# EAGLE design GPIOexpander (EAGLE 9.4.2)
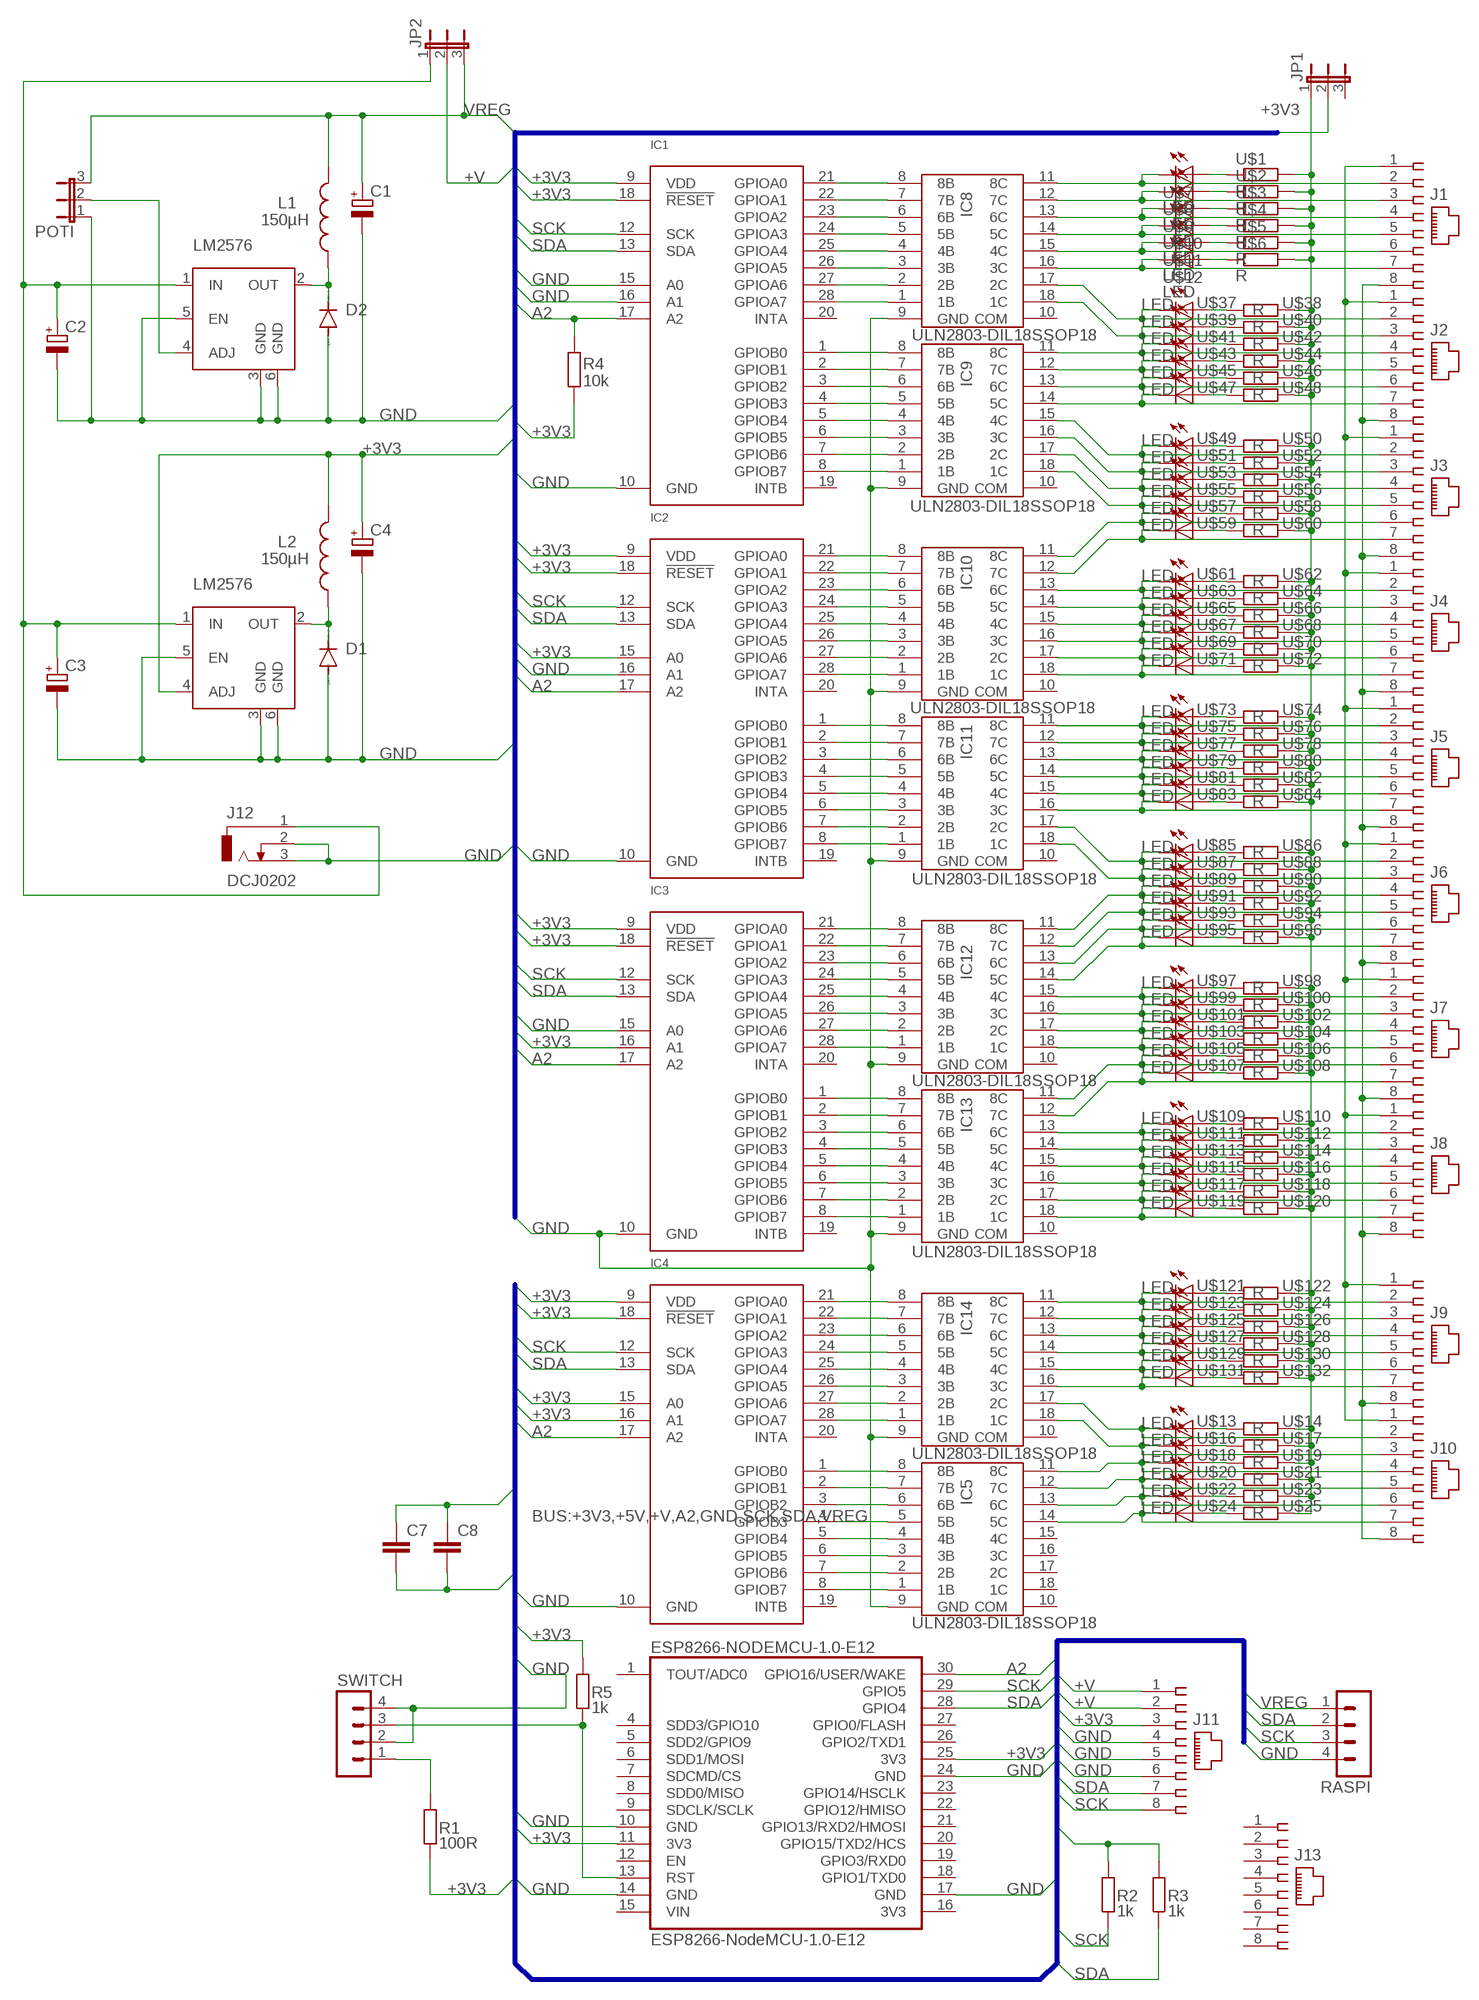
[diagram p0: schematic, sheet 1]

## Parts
C1  CPOL-EUE5-10.5  [E5-10,5]
C2  CPOL-EUE5-10.5  [E5-10,5]
C3  CPOL-EUE5-10.5  [E5-10,5]
C4  CPOL-EUE5-10.5  [E5-10,5]
C7  C-EUC0805  [C0805]
C8  C-EUC0805  [C0805]
D1  DIODE-SMB  [SMB]
D2  DIODE-SMB  [SMB]
ESP8266-NODEMCU-1.0-E12  ESP8266-NodeMCU-1.0-E12  MCP8266-MODULE  [MCP8266-MODULE]
IC1  MCP23017-DIL28-3SSOP28  [SO28W]
IC2  MCP23017-DIL28-3SSOP28  [SO28W]
IC3  MCP23017-DIL28-3SSOP28  [SO28W]
IC4  MCP23017-DIL28-3SSOP28  [SO28W]
IC5  ULN2803-DIL18SSOP18  [SO18W]
IC8  ULN2803-DIL18SSOP18  [SO18W]
IC9  ULN2803-DIL18SSOP18  [SO18W]
IC10  ULN2803-DIL18SSOP18  [SO18W]
IC11  ULN2803-DIL18SSOP18  [SO18W]
IC12  ULN2803-DIL18SSOP18  [SO18W]
IC13  ULN2803-DIL18SSOP18  [SO18W]
IC14  ULN2803-DIL18SSOP18  [SO18W]
J1  215877-7  [215877-7]
J2  215877-7  [215877-7]
J3  215877-7  [215877-7]
J4  215877-7  [215877-7]
J5  215877-7  [215877-7]
J6  215877-7  [215877-7]
J7  215877-7  [215877-7]
J8  215877-7  [215877-7]
J9  215877-7  [215877-7]
J10  215877-7  [215877-7]
J11  215877-7  [215877-7]
J12  DCJ0202  [DCJ0303]
J13  215877-7  [215877-7]
JP1  JP2E  [JP2]
JP2  JP2E  [JP2]
L1  150µH  BIG_COILS  [BIG_COIL]
L2  150µH  BIG_COILS  [BIG_COIL]
POTI  JP2E  [JP2]
R1  100R  R  [C0805]
R2  1k  R  [C0805]
R3  1k  R  [C0805]
R4  10k  R  [C0805]
R5  1k  R  [C0805]
RASPI  MA04-1  [MA04-1]
SWITCH  MA04-1  [MA04-1]
U$1  R  [C0805]
U$2  R  [C0805]
U$3  R  [C0805]
U$4  R  [C0805]
U$5  R  [C0805]
U$6  R  [C0805]
U$7  LED  [C0805]
U$8  LED  [C0805]
U$9  LED  [C0805]
U$10  LED  [C0805]
U$11  LED  [C0805]
U$12  LED  [C0805]
U$13  LED  [C0805]
U$14  R  [C0805]
U$16  LED  [C0805]
U$17  R  [C0805]
U$18  LED  [C0805]
U$19  R  [C0805]
U$20  LED  [C0805]
U$21  R  [C0805]
U$22  LED  [C0805]
U$23  R  [C0805]
U$24  LED  [C0805]
U$25  R  [C0805]
U$26  LM2576  [D2PAK]
U$28  LM2576  [D2PAK]
U$37  LED  [C0805]
U$38  R  [C0805]
U$39  LED  [C0805]
U$40  R  [C0805]
U$41  LED  [C0805]
U$42  R  [C0805]
U$43  LED  [C0805]
U$44  R  [C0805]
U$45  LED  [C0805]
U$46  R  [C0805]
U$47  LED  [C0805]
U$48  R  [C0805]
U$49  LED  [C0805]
U$50  R  [C0805]
U$51  LED  [C0805]
U$52  R  [C0805]
U$53  LED  [C0805]
U$54  R  [C0805]
U$55  LED  [C0805]
U$56  R  [C0805]
U$57  LED  [C0805]
U$58  R  [C0805]
U$59  LED  [C0805]
U$60  R  [C0805]
U$61  LED  [C0805]
U$62  R  [C0805]
U$63  LED  [C0805]
U$64  R  [C0805]
U$65  LED  [C0805]
U$66  R  [C0805]
U$67  LED  [C0805]
U$68  R  [C0805]
U$69  LED  [C0805]
U$70  R  [C0805]
U$71  LED  [C0805]
U$72  R  [C0805]
U$73  LED  [C0805]
U$74  R  [C0805]
U$75  LED  [C0805]
U$76  R  [C0805]
U$77  LED  [C0805]
U$78  R  [C0805]
U$79  LED  [C0805]
U$80  R  [C0805]
U$81  LED  [C0805]
U$82  R  [C0805]
U$83  LED  [C0805]
U$84  R  [C0805]
U$85  LED  [C0805]
U$86  R  [C0805]
U$87  LED  [C0805]
U$88  R  [C0805]
U$89  LED  [C0805]
U$90  R  [C0805]
U$91  LED  [C0805]
U$92  R  [C0805]
U$93  LED  [C0805]
U$94  R  [C0805]
U$95  LED  [C0805]
U$96  R  [C0805]
U$97  LED  [C0805]
U$98  R  [C0805]
U$99  LED  [C0805]
U$100  R  [C0805]
U$101  LED  [C0805]
U$102  R  [C0805]
U$103  LED  [C0805]
U$104  R  [C0805]
U$105  LED  [C0805]
U$106  R  [C0805]
U$107  LED  [C0805]
U$108  R  [C0805]
U$109  LED  [C0805]
U$110  R  [C0805]
U$111  LED  [C0805]
U$112  R  [C0805]
U$113  LED  [C0805]
U$114  R  [C0805]
U$115  LED  [C0805]
U$116  R  [C0805]
U$117  LED  [C0805]
U$118  R  [C0805]
U$119  LED  [C0805]
U$120  R  [C0805]
U$121  LED  [C0805]
U$122  R  [C0805]
U$123  LED  [C0805]
U$124  R  [C0805]
U$125  LED  [C0805]
U$126  R  [C0805]
U$127  LED  [C0805]
U$128  R  [C0805]
U$129  LED  [C0805]
U$130  R  [C0805]
U$131  LED  [C0805]
U$132  R  [C0805]

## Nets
+3V3: C4.+ C7.1 C8.1 ESP8266-NODEMCU-1.0-E12.11(3V3) ESP8266-NODEMCU-1.0-E12.25(3V3) IC1.9(VDD) IC1.18(!RESET) IC2.9(VDD) IC2.15(A0) IC2.18(!RESET) IC3.9(VDD) IC3.16(A1) IC3.18(!RESET) IC4.9(VDD) IC4.15(A0) IC4.16(A1) IC4.18(!RESET) J11.3 JP1.2 L2.P$2 R1.1 R2.2 R3.2 R4.1 R5.2 U$28.4(ADJ)
+V: J1.1 J2.1 J3.1 J4.1 J5.1 J6.1 J7.1 J8.1 J9.1 J10.1 J11.1 J11.2 JP2.2
A2: ESP8266-NODEMCU-1.0-E12.30(GPIO16/USER/WAKE) IC1.17(A2) IC2.17(A2) IC3.17(A2) IC4.17(A2) R4.2
GND: C1.- C2.- C3.- C4.- C7.2 C8.2 D1.A D2.A ESP8266-NODEMCU-1.0-E12.10(GND) ESP8266-NODEMCU-1.0-E12.14(GND) ESP8266-NODEMCU-1.0-E12.17(GND) ESP8266-NODEMCU-1.0-E12.24(GND) IC1.10(GND) IC1.15(A0) IC1.16(A1) IC2.10(GND) IC2.16(A1) IC3.10(GND) IC3.15(A0) IC4.10(GND) IC5.9(GND) IC8.9(GND) IC9.9(GND) IC10.9(GND) IC11.9(GND) IC12.9(GND) IC13.9(GND) IC14.9(GND) J1.8 J2.8 J3.8 J4.8 J5.8 J6.8 J7.8 J8.8 J9.8 J10.8 J11.4 J11.5 J11.6 J12.2 J12.3 POTI.1 RASPI.4 SWITCH.2 SWITCH.4 U$26.3(GND) U$26.5(EN) U$26.6(GND) U$28.3(GND) U$28.5(EN) U$28.6(GND)
N$1: IC1.21(GPIOA0) IC8.8(8B)
N$2: IC1.22(GPIOA1) IC8.7(7B)
N$3: IC1.23(GPIOA2) IC8.6(6B)
N$4: IC1.24(GPIOA3) IC8.5(5B)
N$5: IC1.25(GPIOA4) IC8.4(4B)
N$6: IC1.26(GPIOA5) IC8.3(3B)
N$7: IC1.27(GPIOA6) IC8.2(2B)
N$8: IC1.28(GPIOA7) IC8.1(1B)
N$9: IC4.8(GPIOB7) IC5.1(1B)
N$10: IC1.1(GPIOB0) IC9.8(8B)
N$11: IC1.2(GPIOB1) IC9.7(7B)
N$12: IC1.3(GPIOB2) IC9.6(6B)
N$13: IC1.4(GPIOB3) IC9.5(5B)
N$14: IC1.5(GPIOB4) IC9.4(4B)
N$15: IC1.6(GPIOB5) IC9.3(3B)
N$16: IC1.7(GPIOB6) IC9.2(2B)
N$17: IC1.8(GPIOB7) IC9.1(1B)
N$18: IC4.7(GPIOB6) IC5.2(2B)
N$19: IC2.21(GPIOA0) IC10.8(8B)
N$20: IC2.22(GPIOA1) IC10.7(7B)
N$21: IC2.23(GPIOA2) IC10.6(6B)
N$22: IC2.24(GPIOA3) IC10.5(5B)
N$23: IC2.25(GPIOA4) IC10.4(4B)
N$24: IC2.26(GPIOA5) IC10.3(3B)
N$25: IC2.27(GPIOA6) IC10.2(2B)
N$26: IC2.28(GPIOA7) IC10.1(1B)
N$27: IC4.6(GPIOB5) IC5.3(3B)
N$28: IC2.1(GPIOB0) IC11.8(8B)
N$29: IC2.2(GPIOB1) IC11.7(7B)
N$30: IC2.3(GPIOB2) IC11.6(6B)
N$31: IC2.4(GPIOB3) IC11.5(5B)
N$32: IC2.5(GPIOB4) IC11.4(4B)
N$33: IC2.6(GPIOB5) IC11.3(3B)
N$34: IC2.7(GPIOB6) IC11.2(2B)
N$35: IC2.8(GPIOB7) IC11.1(1B)
N$36: IC9.15(4C) J3.2 U$49.2(C)
N$37: IC3.21(GPIOA0) IC12.8(8B)
N$38: IC3.22(GPIOA1) IC12.7(7B)
N$39: IC3.23(GPIOA2) IC12.6(6B)
N$40: IC3.24(GPIOA3) IC12.5(5B)
N$41: IC3.25(GPIOA4) IC12.4(4B)
N$42: IC3.26(GPIOA5) IC12.3(3B)
N$43: IC3.27(GPIOA6) IC12.2(2B)
N$44: IC3.28(GPIOA7) IC12.1(1B)
N$45: IC9.16(3C) J3.3 U$51.2(C)
N$46: IC3.1(GPIOB0) IC13.8(8B)
N$47: IC3.2(GPIOB1) IC13.7(7B)
N$48: IC3.3(GPIOB2) IC13.6(6B)
N$49: IC3.4(GPIOB3) IC13.5(5B)
N$50: IC3.5(GPIOB4) IC13.4(4B)
N$51: IC3.6(GPIOB5) IC13.3(3B)
N$52: IC3.7(GPIOB6) IC13.2(2B)
N$53: IC3.8(GPIOB7) IC13.1(1B)
N$54: IC9.17(2C) J3.4 U$53.2(C)
N$55: IC4.21(GPIOA0) IC14.8(8B)
N$56: IC4.22(GPIOA1) IC14.7(7B)
N$57: IC4.23(GPIOA2) IC14.6(6B)
N$58: IC4.24(GPIOA3) IC14.5(5B)
N$59: IC4.25(GPIOA4) IC14.4(4B)
N$60: IC4.26(GPIOA5) IC14.3(3B)
N$61: IC4.27(GPIOA6) IC14.2(2B)
N$62: IC4.28(GPIOA7) IC14.1(1B)
N$63: IC8.17(2C) J2.2 U$37.2(C)
N$64: IC4.5(GPIOB4) IC5.4(4B)
N$65: IC4.4(GPIOB3) IC5.5(5B)
N$66: IC4.3(GPIOB2) IC5.6(6B)
N$67: IC4.2(GPIOB1) IC5.7(7B)
N$68: IC4.1(GPIOB0) IC5.8(8B)
N$69: IC14.17(2C) J10.2 U$13.2(C)
N$70: JP1.1 U$1.2 U$2.2 U$3.2 U$4.2 U$5.2 U$6.2 U$14.2 U$17.2 U$19.2 U$21.2 U$23.2 U$25.2 U$38.2 U$40.2 U$42.2 U$44.2 U$46.2 U$48.2 U$50.2 U$52.2 U$54.2 U$56.2 U$58.2 U$60.2 U$62.2 U$64.2 U$66.2 U$68.2 U$70.2 U$72.2 U$74.2 U$76.2 U$78.2 U$80.2 U$82.2 U$84.2 U$86.2 U$88.2 U$90.2 U$92.2 U$94.2 U$96.2 U$98.2 U$100.2 U$102.2 U$104.2 U$106.2 U$108.2 U$110.2 U$112.2 U$114.2 U$116.2 U$118.2 U$120.2 U$122.2 U$124.2 U$126.2 U$128.2 U$130.2 U$132.2
N$71: D2.C L1.P$1 U$26.2(OUT)
N$72: IC8.11(8C) J1.2 U$7.2(C)
N$73: C2.+ C3.+ J12.1 JP2.1 U$26.1(IN) U$28.1(IN)
N$74: IC14.18(1C) J10.3 U$16.2(C)
N$75: IC5.11(8C) J10.4 U$18.2(C)
N$76: IC5.12(7C) J10.5 U$20.2(C)
N$77: IC5.13(6C) J10.6 U$22.2(C)
N$78: IC5.14(5C) J10.7 U$24.2(C)
N$79: U$13.1(A) U$14.1
N$80: U$16.1(A) U$17.1
N$81: IC8.18(1C) J2.3 U$39.2(C)
N$82: U$18.1(A) U$19.1
N$83: U$20.1(A) U$21.1
N$84: U$22.1(A) U$23.1
N$85: U$24.1(A) U$25.1
N$86: POTI.2 U$26.4(ADJ)
N$87: D1.C L2.P$1 U$28.2(OUT)
N$88: ESP8266-NODEMCU-1.0-E12.13(RST) R5.1 SWITCH.3
N$89: R1.2 SWITCH.1
N$90: IC9.12(7C) J2.5 U$43.2(C)
N$99: IC9.11(8C) J2.4 U$41.2(C)
N$128: IC9.18(1C) J3.5 U$55.2(C)
N$215: IC10.11(8C) J3.6 U$57.2(C)
N$217: IC8.12(7C) J1.3 U$8.2(C)
N$218: IC8.13(6C) J1.4 U$9.2(C)
N$223: IC9.13(6C) J2.6 U$45.2(C)
N$224: IC9.14(5C) J2.7 U$47.2(C)
N$225: IC8.14(5C) J1.5 U$10.2(C)
N$226: IC8.15(4C) J1.6 U$11.2(C)
N$228: IC8.16(3C) J1.7 U$12.2(C)
N$229: IC10.12(7C) J3.7 U$59.2(C)
N$230: IC10.13(6C) J4.2 U$61.2(C)
N$232: IC10.14(5C) J4.3 U$63.2(C)
N$233: IC10.15(4C) J4.4 U$65.2(C)
N$234: IC10.16(3C) J4.5 U$67.2(C)
N$235: IC10.17(2C) J4.6 U$69.2(C)
N$238: IC10.18(1C) J4.7 U$71.2(C)
N$239: IC11.14(5C) J5.5 U$79.2(C)
N$240: IC11.15(4C) J5.6 U$81.2(C)
N$241: IC11.16(3C) J5.7 U$83.2(C)
N$242: IC11.11(8C) J5.2 U$73.2(C)
N$243: IC11.12(7C) J5.3 U$75.2(C)
N$244: IC11.13(6C) J5.4 U$77.2(C)
N$245: IC11.17(2C) J6.2 U$85.2(C)
N$246: IC11.18(1C) J6.3 U$87.2(C)
N$247: IC12.11(8C) J6.4 U$89.2(C)
N$248: IC12.12(7C) J6.5 U$91.2(C)
N$249: IC12.13(6C) J6.6 U$93.2(C)
N$250: IC12.14(5C) J6.7 U$95.2(C)
N$251: IC12.15(4C) J7.2 U$97.2(C)
N$252: IC12.16(3C) J7.3 U$99.2(C)
N$253: IC12.17(2C) J7.4 U$101.2(C)
N$254: IC12.18(1C) J7.5 U$103.2(C)
N$255: IC13.11(8C) J7.6 U$105.2(C)
N$256: IC13.12(7C) J7.7 U$107.2(C)
N$257: IC13.13(6C) J8.2 U$109.2(C)
N$258: IC13.14(5C) J8.3 U$111.2(C)
N$259: IC13.15(4C) J8.4 U$113.2(C)
N$260: IC13.16(3C) J8.5 U$115.2(C)
N$261: IC13.17(2C) J8.6 U$117.2(C)
N$262: IC13.18(1C) J8.7 U$119.2(C)
N$263: IC14.11(8C) J9.2 U$121.2(C)
N$264: IC14.12(7C) J9.3 U$123.2(C)
N$265: IC14.13(6C) J9.4 U$125.2(C)
N$266: IC14.14(5C) J9.5 U$127.2(C)
N$267: IC14.15(4C) J9.6 U$129.2(C)
N$268: IC14.16(3C) J9.7 U$131.2(C)
N$329: U$1.1 U$7.1(A)
N$330: U$2.1 U$8.1(A)
N$331: U$3.1 U$9.1(A)
N$332: U$4.1 U$10.1(A)
N$333: U$5.1 U$11.1(A)
N$334: U$6.1 U$12.1(A)
N$347: U$37.1(A) U$38.1
N$348: U$39.1(A) U$40.1
N$349: U$41.1(A) U$42.1
N$350: U$43.1(A) U$44.1
N$351: U$45.1(A) U$46.1
N$352: U$47.1(A) U$48.1
N$353: U$49.1(A) U$50.1
N$354: U$51.1(A) U$52.1
N$355: U$53.1(A) U$54.1
N$356: U$55.1(A) U$56.1
N$357: U$57.1(A) U$58.1
N$358: U$59.1(A) U$60.1
N$359: U$61.1(A) U$62.1
N$360: U$63.1(A) U$64.1
N$361: U$65.1(A) U$66.1
N$362: U$67.1(A) U$68.1
N$363: U$69.1(A) U$70.1
N$364: U$71.1(A) U$72.1
N$365: U$73.1(A) U$74.1
N$366: U$75.1(A) U$76.1
N$367: U$77.1(A) U$78.1
N$368: U$79.1(A) U$80.1
N$369: U$81.1(A) U$82.1
N$370: U$83.1(A) U$84.1
N$371: U$85.1(A) U$86.1
N$372: U$87.1(A) U$88.1
N$373: U$89.1(A) U$90.1
N$374: U$91.1(A) U$92.1
N$375: U$93.1(A) U$94.1
N$376: U$95.1(A) U$96.1
N$377: U$97.1(A) U$98.1
N$378: U$99.1(A) U$100.1
N$379: U$101.1(A) U$102.1
N$380: U$103.1(A) U$104.1
N$381: U$105.1(A) U$106.1
N$382: U$107.1(A) U$108.1
N$383: U$109.1(A) U$110.1
N$384: U$111.1(A) U$112.1
N$385: U$113.1(A) U$114.1
N$386: U$115.1(A) U$116.1
N$387: U$117.1(A) U$118.1
N$388: U$119.1(A) U$120.1
N$389: U$121.1(A) U$122.1
N$390: U$123.1(A) U$124.1
N$391: U$125.1(A) U$126.1
N$392: U$127.1(A) U$128.1
N$393: U$129.1(A) U$130.1
N$394: U$131.1(A) U$132.1
SCK: ESP8266-NODEMCU-1.0-E12.29(GPIO5) IC1.12(SCK) IC2.12(SCK) IC3.12(SCK) IC4.12(SCK) J11.8 R2.1 RASPI.3
SDA: ESP8266-NODEMCU-1.0-E12.28(GPIO4) IC1.13(SDA) IC2.13(SDA) IC3.13(SDA) IC4.13(SDA) J11.7 R3.1 RASPI.2
VREG: C1.+ JP2.3 L1.P$2 POTI.3 RASPI.1
Unconnected: ESP8266-NODEMCU-1.0-E12.1(TOUT/ADC0) ESP8266-NODEMCU-1.0-E12.4(SDD3/GPIO10) ESP8266-NODEMCU-1.0-E12.5(SDD2/GPIO9) ESP8266-NODEMCU-1.0-E12.6(SDD1/MOSI) ESP8266-NODEMCU-1.0-E12.7(SDCMD/CS) ESP8266-NODEMCU-1.0-E12.8(SDD0/MISO) ESP8266-NODEMCU-1.0-E12.9(SDCLK/SCLK) ESP8266-NODEMCU-1.0-E12.12(EN) ESP8266-NODEMCU-1.0-E12.15(VIN) ESP8266-NODEMCU-1.0-E12.16(3V3) ESP8266-NODEMCU-1.0-E12.18(GPIO1/TXD0) ESP8266-NODEMCU-1.0-E12.19(GPIO3/RXD0) ESP8266-NODEMCU-1.0-E12.20(GPIO15/TXD2/HCS) ESP8266-NODEMCU-1.0-E12.21(GPIO13/RXD2/HMOSI) ESP8266-NODEMCU-1.0-E12.22(GPIO12/HMISO) ESP8266-NODEMCU-1.0-E12.23(GPIO14/HSCLK) ESP8266-NODEMCU-1.0-E12.26(GPIO2/TXD1) ESP8266-NODEMCU-1.0-E12.27(GPIO0/FLASH) IC1.19(INTB) IC1.20(INTA) IC2.19(INTB) IC2.20(INTA) IC3.19(INTB) IC3.20(INTA) IC4.19(INTB) IC4.20(INTA) IC5.10(COM) IC5.15(4C) IC5.16(3C) IC5.17(2C) IC5.18(1C) IC8.10(COM) IC9.10(COM) IC10.10(COM) IC11.10(COM) IC12.10(COM) IC13.10(COM) IC14.10(COM) J13.1 J13.2 J13.3 J13.4 J13.5 J13.6 J13.7 J13.8 JP1.3

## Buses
BUS:+3V3,+5V,+V,A2,GND,SCK,SDA,VREG

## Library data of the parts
C1-C4 = rcl:CPOL-EU: POLARIZED CAPACITOR, European symbol; SPICEPREFIX: C
C7 C8 = rcl:C-EU: CAPACITOR, European symbol; SPICEPREFIX: C
D1 D2 = diode:DIODE-: DIODE
ESP8266-NODEMCU-1.0-E12 = GPIOexpander:MCP8266-MODULE
IC1 = GPIOexpander:MCP23017-DIL28-3: GPIO expander; SPICEPREFIX: X
IC2-IC4 = GPIOexpander:MCP23017-DIL28-3: GPIO expander
IC5 IC8-IC14 = GPIOexpander:ULN2803-DIL18
J1-J11 J13 = con-amp:215877-7: AMP connector
J12 = GPIOexpander:DCJ0202: DC POWER JACK Source: DCJ0202.pdf
JP1 JP2 POTI = jumper-alex:JP2E: JUMPER
L1 L2 = GPIOexpander:BIG_COILS
R1-R5 U$1-U$6 U$14 U$17 U$19 U$21 U$23 U$25 U$38 U$40 U$42 U$44 U$46 U$48 U$50 U$52 U$54 U$56 U$58 U$60 U$62 U$64 U$66 U$68 U$70 U$72 U$74 U$76 U$78 U$80 U$82 U$84 U$86 U$88 U$90 U$92 U$94 U$96 U$98 U$100 U$102 U$104 U$106 U$108 U$110 U$112 U$114 U$116 U$118 U$120 U$122 U$124 U$126 U$128 U$130 U$132 = GPIOexpander:R
RASPI SWITCH = con-lstb:MA04-1: PIN HEADER; OC_FARNELL: unknown; OC_NEWARK: unknown
U$7-U$13 U$16 U$18 U$20 U$22 U$24 U$37 U$39 U$41 U$43 U$45 U$47 U$49 U$51 U$53 U$55 U$57 U$59 U$61 U$63 U$65 U$67 U$69 U$71 U$73 U$75 U$77 U$79 U$81 U$83 U$85 U$87 U$89 U$91 U$93 U$95 U$97 U$99 U$101 U$103 U$105 U$107 U$109 U$111 U$113 U$115 U$117 U$119 U$121 U$123 U$125 U$127 U$129 U$131 = GPIOexpander:LED
U$26 U$28 = GPIOexpander:LM2576

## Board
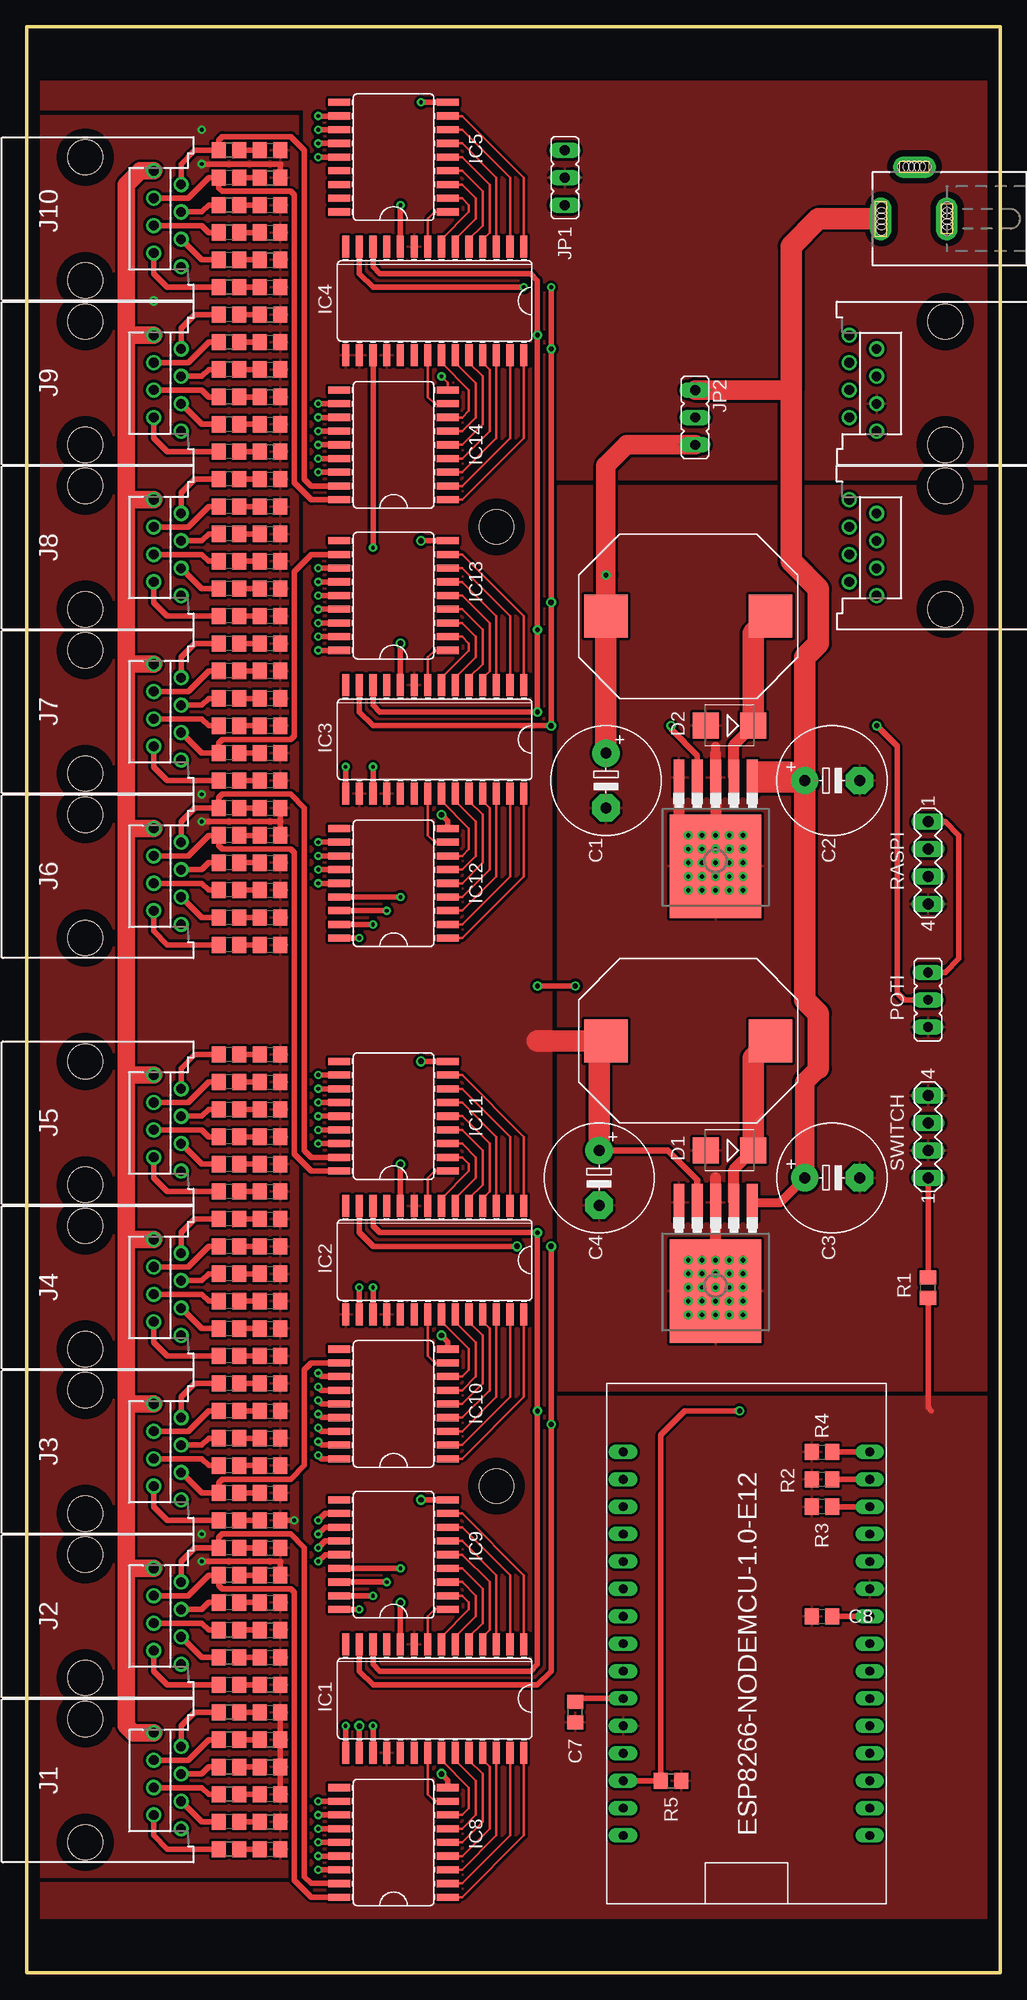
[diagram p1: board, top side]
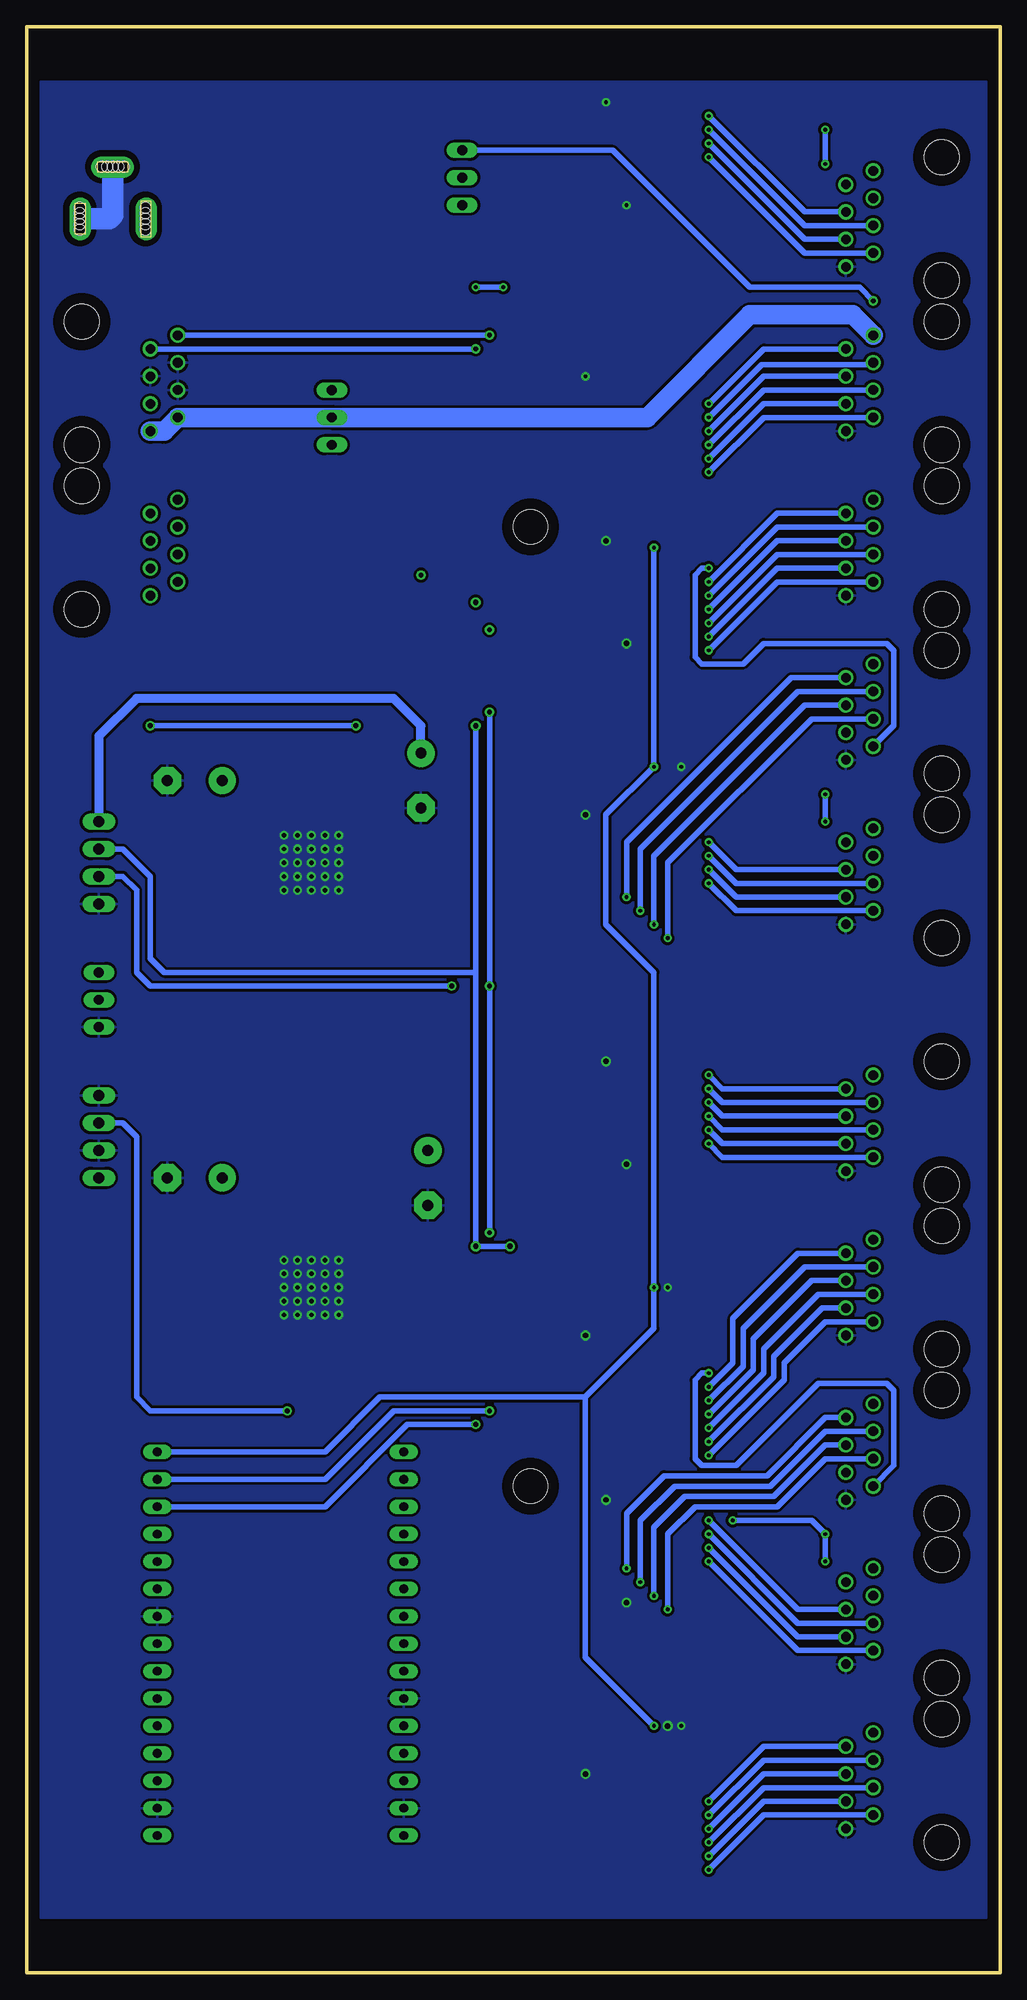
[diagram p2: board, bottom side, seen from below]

Size 90.17 x 180.34 mm. Coordinates in mm from the lower left corner, seen from the top.
Outline: 0,0 90.17,0 90.17,180.34 0,180.34 0,0
Copper layers (1*16): Top 0.035mm / dielectric 1.5mm / Bottom 0.035mm
Design rules "default": minimum track width 6mil, minimum drill 0.35mm, track to track 6mil, track to pad 6mil, pad to pad 6mil, via to via 6mil, smd to smd 6mil, copper to edge 40mil, drill to drill 6mil, minimum pad ring 10mil, minimum via ring 8mil, stop-mask expansion 4mil, vias tented up to drill 0mil, thermal gap 10mil
Holes 3.2 mm at 43.5,133.99 43.5,45.09

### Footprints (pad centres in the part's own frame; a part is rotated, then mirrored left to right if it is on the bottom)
E5-10,5 = drill 1.016 pad 2.54: + -2.54,0 | drill 1.016 pad 2.54 octagon: - 2.54,0
C0805 = smd 1.3 x 1.5: 1 -0.95,0; 2 0.95,0
SMB = smd 2.4 x 2.4: A 2.2,0; C -2.2,0
MCP8266-MODULE = drill 0.813 long: 1 41.91,24.13; 2 39.37,24.13; 3 36.83,24.13; 4 34.29,24.13; 5 31.75,24.13; 6 29.21,24.13; 7 26.67,24.13; 8 24.13,24.13; 9 21.59,24.13; 10 19.05,24.13; 11 16.51,24.13; 12 13.97,24.13; 13 11.43,24.13; 14 8.89,24.13; 15 6.35,24.13; 16 6.35,1.27; 17 8.89,1.27; 18 11.43,1.27; 19 13.97,1.27; 20 16.51,1.27; 21 19.05,1.27; 22 21.59,1.27; 23 24.13,1.27; 24 26.67,1.27; 25 29.21,1.27; 26 31.75,1.27; 27 34.29,1.27; 28 36.83,1.27; 29 39.37,1.27; 30 41.91,1.27
SO28W = smd 0.66 x 2.032: 1 -8.255,-5.029; 2 -6.985,-5.029; 3 -5.715,-5.029; 4 -4.445,-5.029; 5 -3.175,-5.029; 6 -1.905,-5.029; 7 -0.635,-5.029; 8 0.635,-5.029; 9 1.905,-5.029; 10 3.175,-5.029; 11 4.445,-5.029; 12 5.715,-5.029; 13 6.985,-5.029; 14 8.255,-5.029; 15 8.255,5.029; 16 6.985,5.029; 17 5.715,5.029; 18 4.445,5.029; 19 3.175,5.029; 20 1.905,5.029; 21 0.635,5.029; 22 -0.635,5.029; 23 -1.905,5.029; 24 -3.175,5.029; 25 -4.445,5.029; 26 -5.715,5.029; 27 -6.985,5.029; 28 -8.255,5.029
SO18W = smd 0.66 x 2.032: 1 -5.715,-5.029; 2 -4.445,-5.029; 3 -3.175,-5.029; 4 -1.905,-5.029; 5 -0.635,-5.029; 6 0.635,-5.029; 7 1.905,-5.029; 8 3.175,-5.029; 9 4.445,-5.029; 10 4.445,5.029; 11 3.175,5.029; 12 1.905,5.029; 13 0.635,5.029; 14 -0.635,5.029; 15 -1.905,5.029; 16 -3.175,5.029; 17 -4.445,5.029; 18 -5.715,5.029
215877-7 = drill 0.889: 1 -4.445,6.35; 2 -3.175,8.89; 3 -1.905,6.35; 4 -0.635,8.89; 5 0.635,6.35; 6 1.905,8.89; 7 3.175,6.35; 8 4.445,8.89 | hole 3.251: -5.715,0; 5.715,0
DCJ0303 = drill 1 pad 2 long: 1 0,3.1; 2 4.8,0; 3 0,-3 | hole 1: 0,3.048; 0.508,3.048; -0.508,3.048; -1.016,3.048; 1.016,3.048; 0,-3.048; 0.508,-3.048; 1.016,-3.048; -0.508,-3.048; -1.016,-3.048; 4.826,0; 4.826,0.508; 4.826,1.016; 4.826,-0.508; 4.826,-1.016
JP2 = drill 0.914 long: 1 -2.54,0; 2 0,0; 3 2.54,0
BIG_COIL = smd 4 x 4: P$1 15.24,0; P$2 0,0
MA04-1 = drill 1.016 long: 1 -3.81,0; 2 -1.27,0; 3 1.27,0; 4 3.81,0
D2PAK = smd 1 x 3.4: 1 -3.4,-7.875; 2 -1.7,-7.875; 3 0,-7.875; 4 1.7,-7.875; 5 3.4,-7.875 | smd 8.5 x 9.6: 6 0,0.325

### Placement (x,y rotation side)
C1  53.66,110.49 270 top
C2  74.61,110.49 0 top
C3  74.61,73.66 0 top
C4  53.02,73.66 270 top
C7  50.8,24.13 90 top
C8  73.66,33.02 0 top
D1  65.09,76.2 180 top
D2  65.09,115.57 180 top
ESP8266-NODEMCU-1.0-E12  79.38,6.35 90 top
IC1  37.78,25.4 180 top
IC2  37.78,66.04 180 top
IC3  37.78,114.3 180 top
IC4  37.78,154.94 180 top
IC5  33.97,168.91 90 top
IC8  33.97,12.7 90 top
IC9  33.97,39.37 90 top
IC10  33.97,53.34 90 top
IC11  33.97,80.01 90 top
IC12  33.97,101.6 90 top
IC13  33.97,128.27 90 top
IC14  33.97,142.24 90 top
J1  5.4,17.78 270 top
J2  5.4,33.02 270 top
J3  5.4,48.26 270 top
J4  5.4,63.5 270 top
J5  5.4,78.74 270 top
J6  5.4,101.6 270 top
J7  5.4,116.84 270 top
J8  5.4,132.08 270 top
J9  5.4,147.32 270 top
J10  5.4,162.56 270 top
J11  85.09,147.32 90 top
J12  82.23,162.56 90 top
J13  85.09,132.08 90 top
JP1  49.85,166.37 270 top
JP2  61.91,144.15 270 top
L1  53.66,125.73 0 top
L2  53.66,86.36 0 top
POTI  83.5,90.17 90 top
R1  83.5,63.5 90 top
R2  73.66,45.72 180 top
R3  73.66,43.18 180 top
R4  73.66,48.26 0 top
R5  59.69,17.78 0 top
RASPI  83.5,102.87 270 top
SWITCH  83.5,77.47 90 top
U$1  22.54,24.13 0 top
U$2  22.54,21.59 0 top
U$3  22.54,19.05 0 top
U$4  22.54,16.51 0 top
U$5  22.54,13.97 0 top
U$6  22.54,11.43 0 top
U$7  18.73,24.13 180 top
U$8  18.73,21.59 180 top
U$9  18.73,19.05 180 top
U$10  18.73,16.51 180 top
U$11  18.73,13.97 180 top
U$12  18.73,11.43 180 top
U$13  18.73,168.91 180 top
U$14  22.54,168.91 0 top
U$16  18.73,166.37 180 top
U$17  22.54,166.37 0 top
U$18  18.73,163.83 180 top
U$19  22.54,163.83 0 top
U$20  18.73,161.29 180 top
U$21  22.54,161.29 0 top
U$22  18.73,158.75 180 top
U$23  22.54,158.75 0 top
U$24  18.73,156.21 180 top
U$25  22.54,156.21 0 top
U$26  63.82,102.87 180 top
U$28  63.82,63.5 180 top
U$37  18.73,39.37 180 top
U$38  22.54,39.37 0 top
U$39  18.73,36.83 180 top
U$40  22.54,36.83 0 top
U$41  18.73,34.29 180 top
U$42  22.54,34.29 0 top
U$43  18.73,31.75 180 top
U$44  22.54,31.75 0 top
U$45  18.73,29.21 180 top
U$46  22.54,29.21 0 top
U$47  18.73,26.67 180 top
U$48  22.54,26.67 0 top
U$49  18.73,54.61 180 top
U$50  22.54,54.61 0 top
U$51  18.73,52.07 180 top
U$52  22.54,52.07 0 top
U$53  18.73,49.53 180 top
U$54  22.54,49.53 0 top
U$55  18.73,46.99 180 top
U$56  22.54,46.99 0 top
U$57  18.73,44.45 180 top
U$58  22.54,44.45 0 top
U$59  18.73,41.91 180 top
U$60  22.54,41.91 0 top
U$61  18.73,69.85 180 top
U$62  22.54,69.85 0 top
U$63  18.73,67.31 180 top
U$64  22.54,67.31 0 top
U$65  18.73,64.77 180 top
U$66  22.54,64.77 0 top
U$67  18.73,62.23 180 top
U$68  22.54,62.23 0 top
U$69  18.73,59.69 180 top
U$70  22.54,59.69 0 top
U$71  18.73,57.15 180 top
U$72  22.54,57.15 0 top
U$73  18.73,85.09 180 top
U$74  22.54,85.09 0 top
U$75  18.73,82.55 180 top
U$76  22.54,82.55 0 top
U$77  18.73,80.01 180 top
U$78  22.54,80.01 0 top
U$79  18.73,77.47 180 top
U$80  22.54,77.47 0 top
U$81  18.73,74.93 180 top
U$82  22.54,74.93 0 top
U$83  18.73,72.39 180 top
U$84  22.54,72.39 0 top
U$85  18.73,107.95 180 top
U$86  22.54,107.95 0 top
U$87  18.73,105.41 180 top
U$88  22.54,105.41 0 top
U$89  18.73,102.87 180 top
U$90  22.54,102.87 0 top
U$91  18.73,100.33 180 top
U$92  22.54,100.33 0 top
U$93  18.73,97.79 180 top
U$94  22.54,97.79 0 top
U$95  18.73,95.25 180 top
U$96  22.54,95.25 0 top
U$97  18.73,123.19 180 top
U$98  22.54,123.19 0 top
U$99  18.73,120.65 180 top
U$100  22.54,120.65 0 top
U$101  18.73,118.11 180 top
U$102  22.54,118.11 0 top
U$103  18.73,115.57 180 top
U$104  22.54,115.57 0 top
U$105  18.73,113.03 180 top
U$106  22.54,113.03 0 top
U$107  18.73,110.49 180 top
U$108  22.54,110.49 0 top
U$109  18.73,138.43 180 top
U$110  22.54,138.43 0 top
U$111  18.73,135.89 180 top
U$112  22.54,135.89 0 top
U$113  18.73,133.35 180 top
U$114  22.54,133.35 0 top
U$115  18.73,130.81 180 top
U$116  22.54,130.81 0 top
U$117  18.73,128.27 180 top
U$118  22.54,128.27 0 top
U$119  18.73,125.73 180 top
U$120  22.54,125.73 0 top
U$121  18.73,153.67 180 top
U$122  22.54,153.67 0 top
U$123  18.73,151.13 180 top
U$124  22.54,151.13 0 top
U$125  18.73,148.59 180 top
U$126  22.54,148.59 0 top
U$127  18.73,146.05 180 top
U$128  22.54,146.05 0 top
U$129  18.73,143.51 180 top
U$130  22.54,143.51 0 top
U$131  18.73,140.97 180 top
U$132  22.54,140.97 0 top

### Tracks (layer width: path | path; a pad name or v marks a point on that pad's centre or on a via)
+3V3
  Top 0.508: R1.1 83.5,52.39 83.82,52.07
  Top 0.61: U$28.4 62.12,73.45 59.37,76.2 C4.+
  Top 2: 47.31,86.36 L2.P$2 53.02,85.73 C4.+
  pour Top (isolate 0.254): 1.27,5.08 1.27,8.26 25.72,8.26 25.72,172.72 1.27,172.72 1.27,175.26 88.9,175.26 88.9,138.43 48.58,138.43 48.58,53.34 88.9,53.34 88.9,5.08
+V
  Top 1.27: 9.53,67.95 9.21,67.63
  Top 1.6: 9.21,37.47 9.21,52.71 | 9.21,52.71 9.21,67.63 9.21,83.19 | 9.21,83.19 9.21,106.05 | 9.21,106.05 9.21,121.28 | 9.21,121.28 9.21,136.53 | J2.1 9.21,37.47 | J3.1 9.21,52.71 | J4.1 9.53,67.95 | J5.1 9.21,83.19 | J6.1 9.21,106.05 | J7.1 9.21,121.28 | J8.1 9.21,136.53 | J1.1 9.84,22.22 9.21,22.86 9.21,37.47 | J10.1 10.48,167 9.21,165.74 9.21,151.77 | 9.21,136.53 9.21,151.77 | J9.1 9.21,151.77
  Bottom 1.8: J9.1 13.65,153.67 23.18,153.67 32.7,144.15 JP2.2 J11.2 77.47,142.88 J11.1
A2  (via drill 0.35)
  Top 0.508: v32.07,22.86 IC1.17 | IC3.17 v32.07,111.76 | IC2.17 v32.07,63.5 | v32.07,132.08 IC4.17 | R4.2 ESP8266-NODEMCU-1.0-E12.30
  Bottom 0.508: v32.07,22.86 38.42,29.21 38.42,53.34 | v32.07,132.08 v32.07,111.76 36.51,107.31 36.51,97.16 32.07,92.71 v32.07,63.5 32.07,59.69 38.42,53.34 | ESP8266-NODEMCU-1.0-E12.30 62.55,48.26 57.47,53.34 38.42,53.34
GND  (via drill 0.35, 0.4, 0.5)
  Top 0.254: IC14.9 39,147.37 v38.42,147.96
  Top 0.508: IC10.9 39,58.47 v38.42,59.05 | IC11.9 v36.51,84.45 | IC12.9 39,106.73 v38.42,107.31 | IC13.9 v36.51,132.72 | IC2.10 v34.61,74.93 | IC9.9 v36.51,43.82 | IC1.10 v34.61,34.29 | IC8.9 39,17.83 v38.42,18.41 | IC1.16 v30.8,22.86 | IC3.10 v34.61,123.19 | IC4.10 v34.61,163.83 | IC1.15 v29.53,22.86 | IC2.16 v30.8,63.5 | IC3.15 v29.53,111.76 | IC5.9 v36.51,173.35 | C7.2 51.12,25.4 ESP8266-NODEMCU-1.0-E12.10 | C8.2 ESP8266-NODEMCU-1.0-E12.24
  Top 0.813: 63.82,113.03 63.82,113.67
  Top 1.016: U$26.6 U$26.3 63.82,113.03 | U$26.5 60.42,105 v63.82,101.6 | U$28.6 63.82,73.66
  Bottom 2: J12.3 82.55,162.56 82.23,162.88 J12.2
  other vias: 63.82,102.87 62.55,102.87 65.09,102.87 65.09,101.6 62.55,101.6 62.55,104.14 63.82,104.14 65.09,104.14 65.09,100.33 63.82,100.33 62.55,100.33 61.28,100.33 61.28,101.6 61.28,102.87 61.28,104.14 61.28,105.41 62.55,105.41 63.82,105.41 65.09,105.41 66.36,105.41 66.36,104.14 66.36,102.87 66.36,101.6 66.36,100.33 63.82,63.5 61.28,66.04 66.36,66.04 66.36,60.96 61.28,60.96 63.82,60.96 63.82,66.04 66.36,63.5 61.28,63.5 61.28,64.77 61.28,62.23 62.55,60.96 65.09,60.96 66.36,62.23 66.36,64.77 65.09,66.04 62.55,66.04 62.55,64.77 62.55,63.5 62.55,62.23 63.82,62.23 65.09,62.23 65.09,63.5 65.09,64.77 63.82,64.77
  pour Bottom (isolate 0.254): 1.27,5.08 1.27,175.26 88.9,175.26 88.9,5.08
  pour Top (isolate 0.254): 88.9,137.8 49.21,137.8 49.21,53.98 88.9,53.98
N$1
  Top 0.254: IC1.21 37.15,16.51 37.78,15.88 IC8.8
N$2
  Top 0.203: IC1.22 38.42,19.68
  Top 0.254: 38.42,19.68 40.96,17.14 40.96,15.24 40.32,14.61 IC8.7
N$3
  Top 0.203: IC1.23 39.69,19.68
  Top 0.254: 39.69,19.68 41.59,17.78 41.59,14.61 40.32,13.34 IC8.6
N$4
  Top 0.203: IC1.24 40.96,19.68
  Top 0.254: 40.96,19.68 42.23,18.41 42.23,13.97 40.32,12.07 IC8.5
N$5
  Top 0.203: IC1.25 42.23,19.68
  Top 0.254: 42.23,19.68 42.86,19.05 42.86,13.34 40.32,10.79 IC8.4
N$6
  Top 0.254: IC1.26 43.5,12.7 40.32,9.53 IC8.3
N$7
  Top 0.254: IC1.27 44.77,12.7 40.32,8.26 IC8.2
N$8
  Top 0.254: IC1.28 46.04,12.7 40.32,6.98 IC8.1
N$9
  Top 0.254: IC5.1 37.78,163.19 37.15,162.56 IC4.8
N$10
  Top 0.254: IC1.1 46.04,36.83 40.32,42.55 IC9.8
N$11
  Top 0.254: IC1.2 44.77,36.83 40.32,41.28 IC9.7
N$12
  Top 0.254: IC1.3 43.5,36.83 40.32,40.01 IC9.6
N$13
  Top 0.203: IC1.4 42.23,31.11
  Top 0.254: 42.23,31.11 42.86,31.75 42.86,36.2 40.32,38.73 IC9.5
N$14
  Top 0.203: IC1.5 40.96,31.11
  Top 0.254: 40.96,31.11 42.23,32.38 42.23,35.56 40.32,37.47 IC9.4
N$15
  Top 0.203: IC1.6 39.69,31.11
  Top 0.254: 39.69,31.11 41.59,33.02 41.59,34.92 40.32,36.2 IC9.3
N$16
  Top 0.254: IC1.7 38.42,31.11 40.96,33.66 40.96,34.29 40.32,34.92 IC9.2
N$17
  Top 0.254: IC1.8 37.15,33.02 37.78,33.66 IC9.1
N$18
  Top 0.254: IC4.7 38.42,160.66 40.96,163.19 40.96,163.83 40.32,164.47 IC5.2
N$19
  Top 0.254: IC2.21 37.15,57.15 37.78,56.52 IC10.8
N$20
  Top 0.203: IC2.22 38.42,60.33
  Top 0.254: 38.42,60.33 40.96,57.79 40.96,55.88 40.32,55.25 IC10.7
N$21
  Top 0.203: IC2.23 39.69,60.33
  Top 0.254: 39.69,60.33 41.59,58.42 41.59,55.25 40.32,53.98 IC10.6
N$22
  Top 0.203: IC2.24 40.96,60.33
  Top 0.254: 40.96,60.33 42.23,59.05 42.23,54.61 40.32,52.71 IC10.5
N$23
  Top 0.203: IC2.25 42.23,60.33
  Top 0.254: 42.23,60.33 42.86,59.69 42.86,53.98 40.32,51.44 IC10.4
N$24
  Top 0.254: IC2.26 43.5,53.34 40.32,50.16 IC10.3
N$25
  Top 0.254: IC2.27 44.77,53.34 40.32,48.9 IC10.2
N$26
  Top 0.254: IC2.28 46.04,53.34 40.32,47.62 IC10.1
N$27
  Top 0.254: IC4.6 39.69,160.66 41.59,162.56 41.59,164.47 40.32,165.74 IC5.3
N$28
  Top 0.254: IC2.1 46.04,77.47 40.32,83.19 IC11.8
N$29
  Top 0.254: IC2.2 44.77,77.47 40.32,81.92 IC11.7
N$30
  Top 0.254: IC2.3 43.5,77.47 40.32,80.64 IC11.6
N$31
  Top 0.203: IC2.4 42.23,71.75
  Top 0.254: 42.23,71.75 42.86,72.39 42.86,76.84 40.32,79.38 IC11.5
N$32
  Top 0.203: IC2.5 40.96,71.75
  Top 0.254: 40.96,71.75 42.23,73.03 42.23,76.2 40.32,78.11 IC11.4
N$33
  Top 0.203: IC2.6 39.69,71.75
  Top 0.254: 39.69,71.75 41.59,73.66 41.59,75.56 40.32,76.84 IC11.3
N$34
  Top 0.203: IC2.7 38.42,71.75
  Top 0.254: 38.42,71.75 40.96,74.3 40.96,74.93 40.32,75.56 IC11.2
N$35
  Top 0.254: IC2.8 37.15,73.66 37.78,74.3 IC11.1
N$36  (via drill 0.35)
  Top 0.508: J3.2 14.29,53.34 15.56,54.61 U$49.2 | IC9.15 v34.61,37.47
  Bottom 0.508: v34.61,37.47 34.61,42.55 31.11,46.04 21.59,46.04 16.19,51.44 J3.2
N$37
  Top 0.254: IC3.21 37.15,105.41 37.78,104.78 IC12.8
N$38
  Top 0.203: IC3.22 38.42,108.59
  Top 0.254: 38.42,108.59 40.96,106.05 40.96,104.14 40.32,103.5 IC12.7
N$39
  Top 0.203: IC3.23 39.69,108.59
  Top 0.254: 39.69,108.59 41.59,106.68 41.59,103.5 40.32,102.23 IC12.6
N$40
  Top 0.203: IC3.24 40.96,108.59
  Top 0.254: 40.96,108.59 42.23,107.31 42.23,102.87 40.32,100.97 IC12.5
N$41
  Top 0.203: IC3.25 42.23,108.59
  Top 0.254: 42.23,108.59 42.86,107.95 42.86,102.23 40.32,99.7 IC12.4
N$42
  Top 0.254: IC3.26 43.5,101.6 40.32,98.42 IC12.3
N$43
  Top 0.254: IC3.27 44.77,101.6 40.32,97.16 IC12.2
N$44
  Top 0.254: IC3.28 46.04,101.6 40.32,95.89 IC12.1
N$45  (via drill 0.35)
  Top 0.508: U$51.2 16.83,52.07 14.92,50.16 J3.3 | IC9.16 v33.34,36.2
  Bottom 0.508: v33.34,36.2 33.34,41.91 30.16,45.09 21.27,45.09 16.19,50.16 J3.3
N$46
  Top 0.254: IC3.1 46.04,125.73 40.32,131.44 IC13.8
N$47
  Top 0.254: IC3.2 44.77,125.73 40.32,130.17 IC13.7
N$48
  Top 0.254: IC3.3 43.5,125.73 40.32,128.91 IC13.6
N$49
  Top 0.203: IC3.4 42.23,120.02
  Top 0.254: 42.23,120.02 42.86,120.65 42.86,125.09 40.32,127.64 IC13.5
N$50
  Top 0.203: IC3.5 40.96,120.02
  Top 0.254: 40.96,120.02 42.23,121.28 42.23,124.46 40.32,126.37 IC13.4
N$51
  Top 0.203: IC3.6 39.69,120.02
  Top 0.254: 39.69,120.02 41.59,121.92 41.59,123.83 40.32,125.09 IC13.3
N$52
  Top 0.203: IC3.7 38.42,120.02
  Top 0.254: 38.42,120.02 40.96,122.56 40.96,123.19 40.32,123.83 IC13.2
N$53
  Top 0.254: IC3.8 37.15,121.92 37.78,122.56 IC13.1
N$54  (via drill 0.35)
  Top 0.508: U$53.2 16.83,49.53 16.19,48.9 J3.4 | IC9.17 v32.07,34.92
  Bottom 0.508: v32.07,34.92 32.07,41.28 29.21,44.13 20.95,44.13 16.19,48.9 J3.4
N$55
  Top 0.254: IC4.21 37.15,146.05 37.78,145.41 IC14.8
N$56
  Top 0.254: IC4.22 38.42,149.22 40.96,146.69 40.96,144.78 40.32,144.15 IC14.7
N$57
  Top 0.254: IC4.23 39.69,149.22 41.59,147.32 41.59,144.15 40.32,142.88 IC14.6
N$58
  Top 0.254: IC4.24 40.96,149.22 42.23,147.96 42.23,143.51 40.32,141.6 IC14.5
N$59
  Top 0.254: IC4.25 42.23,149.22 42.86,148.59 42.86,142.88 40.32,140.34 IC14.4
N$60
  Top 0.254: IC4.26 43.5,142.24 40.32,139.06 IC14.3
N$61
  Top 0.254: IC4.27 44.77,142.24 40.32,137.8 IC14.2
N$62
  Top 0.254: IC4.28 46.04,142.24 40.32,136.53 IC14.1
N$63
  Top 0.508: J2.2 14.29,38.1 15.56,39.37 U$37.2 17.78,40.33 18.1,40.64 24.45,40.64 25.72,39.37 25.72,8.89 26.35,8.26 IC8.17
N$64
  Top 0.254: IC4.5 40.96,160.66 42.23,161.93 42.23,165.1 40.32,167 IC5.4
N$65
  Top 0.254: IC4.4 42.23,160.66 42.86,161.29 42.86,165.74 40.32,168.28 IC5.5
N$66
  Top 0.254: IC4.3 43.5,166.37 40.32,169.55 IC5.6
N$67
  Top 0.254: IC5.7 40.32,170.81 44.77,166.37 IC4.2
N$68
  Top 0.254: IC4.1 46.04,166.37 40.32,172.09 IC5.8
N$69
  Top 0.508: J10.2 14.29,167.64 15.56,168.91 U$13.2 17.78,169.87 18.1,170.18 24.45,170.18 25.72,168.91 25.72,138.43 26.35,137.8 IC14.17
N$70  (via drill 0.35, 0.45)
  Top 0.508: U$4.2 U$3.2 U$2.2 U$1.2 | U$88.2 23.49,106.68 | 23.49,106.68 23.5,106.68 | U$40.2 23.49,38.1 23.5,38.1 v16.19,38.1 | U$60.2 v24.77,41.91 | U$17.2 23.49,167.64 23.5,167.64 v16.19,167.64 | U$86.2 23.49,106.68 | 23.49,106.68 v16.19,106.68
  Bottom 0.508: v16.19,38.1 v16.19,40.64 17.46,41.91 v24.77,41.91 | v16.19,167.64 v16.19,170.81 | v16.19,106.68 v16.19,109.22 | v11.75,154.94 13.02,156.21 23.18,156.21 35.88,168.91 JP1.1
  pour Top (isolate 0.254): 25.08,8.89 1.27,8.89 1.27,172.09 25.08,172.09
N$71
  Top 1.016: U$26.2 65.52,113.8 D2.C
  Top 2: D2.C 67.29,124.14 68.88,125.73 L1.P$1
N$72  (via drill 0.35)
  Top 0.508: J1.2 14.29,22.86 15.56,24.13 U$7.2 | IC8.11 v26.99,15.88
  Bottom 0.508: v26.99,15.88 21.91,20.95 J1.2
N$73
  Top 0.813: U$28.1 69.79,71.38 C3.+
  Top 1.016: U$26.1 71.82,110.75 C2.+ | C2.+ 71.44,109.86 67.63,109.86 | C2.+ 70.8,111.76 67.31,111.76
  Top 1.8: C3.+ 72.07,82.55 73.34,83.82 | JP2.1 70.8,146.69
  Top 2: 73.34,83.82 73.34,88.9 72.07,90.17 C2.+ 72.07,121.92 73.34,123.19 73.34,128.27 70.8,130.81 70.8,146.69 70.8,160.02 73.34,162.56 J12.1
N$74
  Top 0.508: J10.3 14.92,164.47 16.83,166.37 U$16.2 17.78,165.41 18.1,165.1 24.45,165.1 24.77,164.78 24.77,138.11 26.35,136.53 IC14.18
N$75  (via drill 0.35)
  Top 0.508: U$18.2 16.83,163.83 16.19,163.19 J10.4 | IC5.11 v26.99,172.09
  Bottom 0.508: v26.99,172.09 18.1,163.19 J10.4
N$76  (via drill 0.35)
  Top 0.508: U$20.2 16.83,161.29 16.19,161.93 J10.5 | IC5.12 v26.99,170.81
  Bottom 0.508: v26.99,170.81 18.1,161.93 J10.5
N$77  (via drill 0.35)
  Top 0.508: U$22.2 16.19,158.75 J10.6 | IC5.13 v26.99,169.55
  Bottom 0.508: v26.99,169.55 18.1,160.66 J10.6
N$78  (via drill 0.35)
  Top 0.508: U$24.2 13.02,156.21 11.75,157.48 J10.7 | IC5.14 v26.99,168.28
  Bottom 0.508: v26.99,168.28 18.1,159.38 J10.7
N$79
  Top 0.508: U$13.1 U$14.1
N$80
  Top 0.508: U$16.1 U$17.1
N$81
  Top 0.508: J2.3 14.92,34.92 16.83,36.83 U$39.2 17.78,35.88 18.1,35.56 24.45,35.56 24.77,35.24 24.77,8.57 26.35,6.98 IC8.18
N$82
  Top 0.508: U$18.1 U$19.1
N$83
  Top 0.508: U$20.1 U$21.1
N$84
  Top 0.508: U$22.1 U$23.1
N$85
  Top 0.508: U$24.1 U$25.1
N$86  (via drill 0.45)
  Top 0.508: U$26.4 62.12,112.83 59.69,115.25 v59.69,115.57 | POTI.2 81.28,90.17 80.64,90.81 80.64,113.67 v78.74,115.57
  Bottom 0.508: v78.74,115.57 v59.69,115.57
N$87
  Top 1.016: U$28.2 65.52,74.43 D1.C
  Top 2: D1.C 67.29,84.75 L2.P$1
N$88  (via drill 0.45)
  Top 0.508: ESP8266-NODEMCU-1.0-E12.13 R5.1 58.74,49.85 60.96,52.07 v66.04,52.07
  Bottom 0.508: v66.04,52.07 78.74,52.07 80.01,53.34 80.01,77.47 81.28,78.74 SWITCH.3
N$89
  Top 0.508: R1.2 SWITCH.1
N$90  (via drill 0.35)
  Top 0.508: U$43.2 16.83,31.75 16.19,32.38 J2.5 | IC9.12 27.62,41.28 v26.99,40.64
  Bottom 0.508: v26.99,40.64 18.73,32.38 J2.5
N$99  (via drill 0.35)
  Top 0.508: U$41.2 16.83,34.29 16.19,33.66 J2.4 | IC9.11 27.62,42.55 v26.99,41.91
  Bottom 0.508: v26.99,41.91 18.73,33.66 J2.4
N$128  (via drill 0.35)
  Top 0.508: U$55.2 16.83,46.99 16.19,47.62 J3.5 | IC9.18 v30.8,33.66
  Bottom 0.508: v30.8,33.66 30.8,40.64 28.26,43.18 20.64,43.18 16.19,47.62 J3.5
N$215
  Top 0.508: J3.6 16.19,44.45 U$57.2 17.78,45.41 18.1,45.72 24.45,45.72 25.72,46.99 25.72,55.88 26.35,56.52 IC10.11
N$217  (via drill 0.35)
  Top 0.508: U$8.2 16.83,21.59 14.92,19.68 J1.3 | IC8.12 v26.99,14.61
  Bottom 0.508: v26.99,14.61 21.91,19.68 J1.3
N$218  (via drill 0.35)
  Top 0.508: U$9.2 16.83,19.05 16.19,18.41 J1.4 | IC8.13 v26.99,13.34
  Bottom 0.508: v26.99,13.34 21.91,18.41 J1.4
N$223  (via drill 0.35)
  Top 0.508: U$45.2 16.19,29.21 J2.6 | IC9.13 27.62,40.01 v26.99,39.37
  Bottom 0.508: v26.99,39.37 18.73,31.11 J2.6
N$224  (via drill 0.35)
  Top 0.508: U$47.2 13.02,26.67 11.75,27.94 J2.7 | IC9.14 27.62,38.73 v26.99,38.1
  Bottom 0.508: v26.99,38.1 18.73,29.84 J2.7
N$225  (via drill 0.35)
  Top 0.508: J1.5 16.19,17.14 16.83,16.51 U$10.2 | IC8.14 v26.99,12.07
  Bottom 0.508: v26.99,12.07 21.91,17.14 J1.5
N$226  (via drill 0.35)
  Top 0.508: U$11.2 16.19,13.97 J1.6 | IC8.15 v26.99,10.79
  Bottom 0.508: v26.99,10.79 21.91,15.88 J1.6
N$228  (via drill 0.35)
  Top 0.508: U$12.2 13.02,11.43 11.75,12.7 J1.7 | IC8.16 v26.99,9.53
  Bottom 0.508: v26.99,9.53 21.91,14.61 J1.7
N$229  (via drill 0.35)
  Top 0.508: U$59.2 13.02,41.91 11.75,43.18 J3.7 | IC10.12 27.3,55.25 v26.99,55.56
  Bottom 0.508: v26.99,55.56 27.62,55.56 28.26,54.93 28.26,47.62 27.62,46.99 24.45,46.99 16.83,54.61 10.48,54.61 9.84,53.98 9.84,46.99 J3.7
N$230  (via drill 0.35)
  Top 0.508: J4.2 14.29,68.58 15.56,69.85 U$61.2 | IC10.13 27.3,53.98 v26.99,54.29
  Bottom 0.508: v26.99,54.29 24.77,56.52 24.77,60.64 18.73,66.67 J4.2
N$232  (via drill 0.35)
  Top 0.508: U$63.2 16.83,67.31 14.92,65.41 J4.3 | IC10.14 27.3,52.71 v26.99,53.02
  Bottom 0.508: v26.99,53.02 23.81,56.2 23.81,59.69 18.1,65.41 J4.3
N$233  (via drill 0.35)
  Top 0.508: U$65.2 16.83,64.77 16.19,64.14 J4.4 | IC10.15 27.3,51.44 v26.99,51.75
  Bottom 0.508: v26.99,51.75 22.86,55.88 22.86,58.74 17.46,64.14 J4.4
N$234  (via drill 0.35)
  Top 0.508: U$67.2 16.83,62.23 16.19,62.87 J4.5 | IC10.16 27.3,50.16 v26.99,50.48
  Bottom 0.508: v26.99,50.48 21.91,55.56 21.91,57.79 16.83,62.87 J4.5
N$235  (via drill 0.35)
  Top 0.508: U$69.2 16.19,59.69 J4.6 | IC10.17 27.3,48.9 v26.99,49.21
  Bottom 0.508: v26.99,49.21 20.98,55.22 20.98,57.11 16.47,61.62 14.31,61.62 J4.6
N$238  (via drill 0.35)
  Top 0.508: U$71.2 13.02,57.15 11.75,58.42 J4.7 | IC10.18 27.3,47.62 v26.99,47.94
  Bottom 0.508: v26.99,47.94 20,54.93 20,56.52 16.19,60.33 J4.7
N$239  (via drill 0.35)
  Top 0.508: U$79.2 16.83,77.47 16.19,78.11 J5.5 | IC11.14 v26.99,79.38
  Bottom 0.508: v26.99,79.38 25.72,78.11 J5.5
N$240  (via drill 0.35)
  Top 0.508: U$81.2 16.19,74.93 J5.6 | IC11.15 v26.99,78.11
  Bottom 0.508: v26.99,78.11 25.72,76.84 J5.6
N$241  (via drill 0.35)
  Top 0.508: U$83.2 13.02,72.39 11.75,73.66 J5.7 | IC11.16 v26.99,76.84
  Bottom 0.508: v26.99,76.84 25.72,75.56 J5.7
N$242  (via drill 0.35)
  Top 0.508: J5.2 14.29,83.82 15.56,85.09 U$73.2 | IC11.11 v26.99,83.19
  Bottom 0.508: v26.99,83.19 25.72,81.92 J5.2
N$243  (via drill 0.35)
  Top 0.508: U$75.2 16.83,82.55 14.92,80.64 J5.3 | IC11.12 v26.99,81.92
  Bottom 0.508: v26.99,81.92 25.72,80.64 J5.3
N$244  (via drill 0.35)
  Top 0.508: U$77.2 16.83,80.01 16.19,79.38 J5.4 | IC11.13 v26.99,80.64
  Bottom 0.508: v26.99,80.64 25.72,79.38 J5.4
N$245
  Top 0.508: J6.2 14.29,106.68 15.56,107.95 U$85.2 17.78,108.91 18.1,109.22 24.45,109.22 25.72,107.95 25.72,76.2 26.35,75.56 IC11.17
N$246
  Top 0.508: J6.3 14.92,103.5 16.83,105.41 U$87.2 17.78,104.45 18.1,104.14 24.45,104.14 24.77,103.82 24.77,75.88 26.35,74.3 IC11.18
N$247  (via drill 0.35)
  Top 0.508: U$89.2 16.83,102.87 16.19,102.23 J6.4 | IC12.11 v26.99,104.78
  Bottom 0.508: v26.99,104.78 24.45,102.23 J6.4
N$248  (via drill 0.35)
  Top 0.508: U$91.2 16.83,100.33 16.19,100.97 J6.5 | IC12.12 v26.99,103.5
  Bottom 0.508: v26.99,103.5 24.45,100.97 J6.5
N$249  (via drill 0.35)
  Top 0.508: U$93.2 16.19,97.79 J6.6 | IC12.13 v26.99,102.23
  Bottom 0.508: v26.99,102.23 24.45,99.7 J6.6
N$250  (via drill 0.35)
  Top 0.508: U$95.2 13.02,95.25 11.75,96.52 J6.7 | IC12.14 v26.99,100.97
  Bottom 0.508: v26.99,100.97 24.45,98.42 J6.7
N$251  (via drill 0.35)
  Top 0.508: J7.2 14.29,121.92 15.56,123.19 U$97.2 | IC12.15 v34.61,99.7
  Bottom 0.508: v34.61,99.7 34.61,104.78 19.37,120.02 J7.2
N$252  (via drill 0.35)
  Top 0.508: U$99.2 16.83,120.65 14.92,118.75 J7.3 | IC12.16 v33.34,98.42
  Bottom 0.508: J7.3 18.73,118.75 33.34,104.14 v33.34,98.42
N$253  (via drill 0.35)
  Top 0.508: U$101.2 16.83,118.11 16.19,117.48 J7.4 | IC12.17 v32.07,97.16
  Bottom 0.508: v32.07,97.16 32.07,103.5 18.1,117.48 J7.4
N$254  (via drill 0.35)
  Top 0.508: U$103.2 16.83,115.57 16.19,116.2 J7.5 | IC12.18 v30.8,95.89
  Bottom 0.508: v30.8,95.89 30.8,102.87 17.46,116.2 J7.5
N$255
  Top 0.508: J7.6 16.19,113.03 U$105.2 17.78,113.98 18.1,114.3 24.45,114.3 24.77,114.62 24.77,129.86 26.35,131.44 IC13.11
N$256  (via drill 0.35)
  Top 0.508: U$107.2 13.02,110.49 11.75,111.76 J7.7 | IC13.12 v26.99,130.17
  Bottom 0.508: J7.7 9.84,115.57 9.84,122.56 10.48,123.19 21.91,123.19 23.81,121.28 27.62,121.28 28.26,121.92 28.26,129.54 27.62,130.17 v26.99,130.17
N$257  (via drill 0.35)
  Top 0.508: J8.2 14.29,137.16 15.56,138.43 U$109.2 | IC13.13 v26.99,128.91
  Bottom 0.508: v26.99,128.91 20.64,135.25 J8.2
N$258  (via drill 0.35)
  Top 0.508: U$111.2 16.83,135.89 14.92,133.99 J8.3 | IC13.14 v26.99,127.64
  Bottom 0.508: v26.99,127.64 20.64,133.99 J8.3
N$259  (via drill 0.35)
  Top 0.508: U$113.2 16.83,133.35 16.19,132.72 J8.4 | IC13.15 v26.99,126.37
  Bottom 0.508: v26.99,126.37 20.64,132.72 J8.4
N$260  (via drill 0.35)
  Top 0.508: U$115.2 16.83,130.81 16.19,131.44 J8.5 | IC13.16 v26.99,125.09
  Bottom 0.508: v26.99,125.09 20.64,131.44 J8.5
N$261  (via drill 0.35)
  Top 0.508: U$117.2 16.19,128.27 J8.6 | IC13.17 v26.99,123.83
  Bottom 0.508: v26.99,123.83 20.64,130.17 J8.6
N$262  (via drill 0.35)
  Top 0.508: U$119.2 13.02,125.73 11.75,127 J8.7 | IC13.18 v26.99,122.56
  Bottom 0.508: v26.99,122.56 20.64,128.91 J8.7
N$263  (via drill 0.35)
  Top 0.508: J9.2 14.29,152.4 15.56,153.67 U$121.2 | IC14.11 v26.99,145.41
  Bottom 0.508: v26.99,145.41 26.95,145.41 21.87,150.5 J9.2
N$264  (via drill 0.35)
  Top 0.508: U$123.2 16.83,151.13 14.92,149.22 J9.3 | IC14.12 v26.99,144.15
  Bottom 0.508: v26.99,144.15 22.07,149.06 11.91,149.06 J9.3
N$265  (via drill 0.35)
  Top 0.508: U$125.2 16.83,148.59 16.19,147.96 J9.4 | IC14.13 v26.99,142.88
  Bottom 0.508: v26.99,142.88 21.91,147.96 J9.4
N$266  (via drill 0.35)
  Top 0.508: U$127.2 16.83,146.05 16.19,146.69 J9.5 | IC14.14 v26.99,141.6
  Bottom 0.508: v26.99,141.6 21.91,146.69 J9.5
N$267  (via drill 0.35)
  Top 0.508: U$129.2 16.19,143.51 J9.6 | IC14.15 v26.99,140.34
  Bottom 0.508: J9.6 21.91,145.41 v26.99,140.34
N$268  (via drill 0.35)
  Top 0.508: U$131.2 13.02,140.97 11.75,142.24 J9.7 | IC14.16 v26.99,139.06
  Bottom 0.508: v26.99,139.06 21.91,144.15 J9.7
N$329
  Top 0.508: U$7.1 U$1.1
N$330
  Top 0.508: U$8.1 U$2.1
N$331
  Top 0.508: U$9.1 U$3.1
N$332
  Top 0.508: U$10.1 U$4.1
N$333
  Top 0.508: U$11.1 U$5.1
N$334
  Top 0.508: U$12.1 U$6.1
N$347
  Top 0.508: U$37.1 U$38.1
N$348
  Top 0.508: U$39.1 U$40.1
N$349
  Top 0.508: U$41.1 U$42.1
N$350
  Top 0.508: U$43.1 U$44.1
N$351
  Top 0.508: U$45.1 U$46.1
N$352
  Top 0.508: U$47.1 U$48.1
N$353
  Top 0.508: U$49.1 U$50.1
N$354
  Top 0.508: U$51.1 U$52.1
N$355
  Top 0.508: U$53.1 U$54.1
N$356
  Top 0.508: U$55.1 U$56.1
N$357
  Top 0.508: U$57.1 U$58.1
N$358
  Top 0.508: U$59.1 U$60.1
N$359
  Top 0.508: U$61.1 U$62.1
N$360
  Top 0.508: U$63.1 U$64.1
N$361
  Top 0.508: U$65.1 U$66.1
N$362
  Top 0.508: U$67.1 U$68.1
N$363
  Top 0.508: U$69.1 U$70.1
N$364
  Top 0.508: U$71.1 U$72.1
N$365
  Top 0.508: U$73.1 U$74.1
N$366
  Top 0.508: U$75.1 U$76.1
N$367
  Top 0.508: U$77.1 U$78.1
N$368
  Top 0.508: U$79.1 U$80.1
N$369
  Top 0.508: U$81.1 U$82.1
N$370
  Top 0.508: U$83.1 U$84.1
N$371
  Top 0.508: U$85.1 U$86.1
N$372
  Top 0.508: U$87.1 U$88.1
N$373
  Top 0.508: U$89.1 U$90.1
N$374
  Top 0.508: U$91.1 U$92.1
N$375
  Top 0.508: U$93.1 U$94.1
N$376
  Top 0.508: U$95.1 U$96.1
N$377
  Top 0.508: U$97.1 U$98.1
N$378
  Top 0.508: U$99.1 U$100.1
N$379
  Top 0.508: U$101.1 U$102.1
N$380
  Top 0.508: U$103.1 U$104.1
N$381
  Top 0.508: U$105.1 U$106.1
N$382
  Top 0.508: U$107.1 U$108.1
N$383
  Top 0.508: U$110.1 U$109.1
N$384
  Top 0.508: U$111.1 U$112.1
N$385
  Top 0.508: U$113.1 U$114.1
N$386
  Top 0.508: U$115.1 U$116.1
N$387
  Top 0.508: U$117.1 U$118.1
N$388
  Top 0.508: U$119.1 U$120.1
N$389
  Top 0.508: U$122.1 U$121.1
N$390
  Top 0.508: U$124.1 U$123.1
N$391
  Top 0.508: U$126.1 U$125.1
N$392
  Top 0.508: U$128.1 U$127.1
N$393
  Top 0.508: U$130.1 U$129.1
N$394
  Top 0.508: U$132.1 U$131.1
SCK  (via drill 0.45)
  Top 0.508: IC2.12 32.07,69.22 32.7,68.58 v47.31,68.58 v47.31,52.07 47.31,28.57 46.67,27.94 32.7,27.94 32.07,28.57 IC1.12 | IC3.12 32.07,117.48 32.7,116.84 v47.31,116.84 v47.31,124.46 v47.31,151.77 47.31,156.84 46.67,157.48 32.7,157.48 32.07,158.12 IC4.12 | ESP8266-NODEMCU-1.0-E12.29 R2.1 | v50.8,91.44 v47.31,91.44
  Bottom 0.508: v47.31,52.07 56.2,52.07 62.55,45.72 ESP8266-NODEMCU-1.0-E12.29 | v47.31,68.58 v47.31,91.44 v47.31,116.84 | J11.8 v47.31,151.77 | v50.8,91.44 78.74,91.44 80.01,92.71 80.01,100.33 81.28,101.6 RASPI.3
SDA  (via drill 0.35, 0.45, 0.5)
  Top 0.508: IC2.13 30.8,68.6 32.09,67.31 v45.4,67.31 | IC3.13 30.8,116.84 32.07,115.57 v48.58,115.57 v48.58,127 v48.58,150.5 v48.58,156.21 | IC1.13 30.8,27.94 32.07,26.67 47.31,26.67 48.58,27.94 v48.58,50.8 v48.58,67.31 | IC4.13 30.8,157.48 32.07,156.21 v46.04,156.21 | ESP8266-NODEMCU-1.0-E12.28 R3.1
  Bottom 0.508: v45.4,67.31 v48.58,67.31 48.58,92.71 | v46.04,156.21 v48.58,156.21 | v48.58,50.8 54.93,50.8 62.55,43.18 ESP8266-NODEMCU-1.0-E12.28 | 48.58,92.71 v48.58,115.57 | J11.7 v48.58,150.5 | 48.58,92.71 77.47,92.71 78.74,93.98 78.74,101.6 81.28,104.14 RASPI.2
VREG  (via drill 0.45)
  Top 0.508: POTI.3 85.09,92.71 86.36,93.98 86.36,105.41 85.09,106.68 RASPI.1
  Top 1.8: L1.P$2 v53.66,129.54 53.66,139.7 55.56,141.6 JP2.3
  Top 2: L1.P$2 C1.+
  Bottom 0.813: C1.+ 53.66,115.57 56.2,118.11 80.01,118.11 83.5,114.62 RASPI.1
